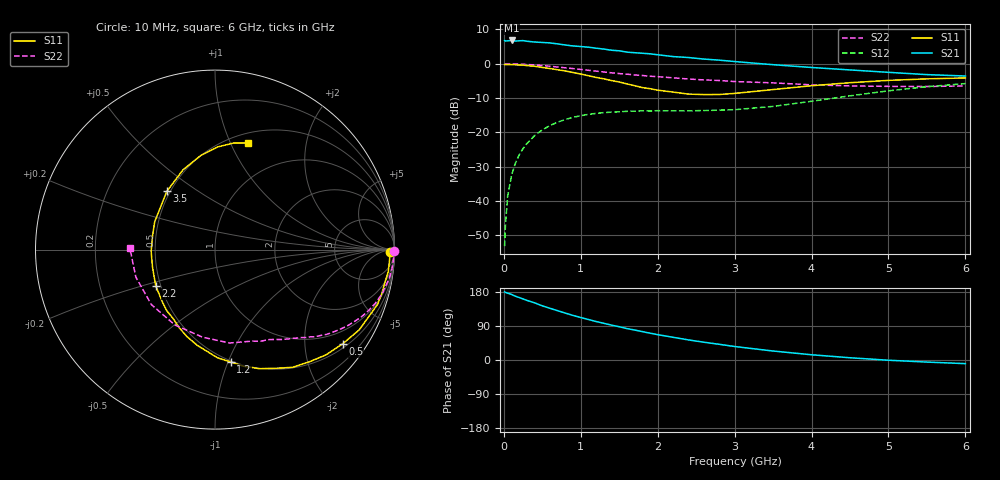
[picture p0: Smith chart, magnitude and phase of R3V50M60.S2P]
! SIEMENS Small Signal Semiconductors
! BFR181
! Si NPN RF Bipolar Junction Transistor in SOT23
! VCE = 0.5 V  IC = 0.6 mA
! Common Emitter S-Parameters:  May  1996
# GHz  S  MA  R  50
!  f  S11  S21  S12  S22
! GHz  MAG  ANG  MAG  ANG  MAG  ANG  MAG  ANG
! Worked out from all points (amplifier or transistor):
!   36 points, 10 MHz to 6 GHz, reference 50 ohm
!   highest |S21| = 6.8 dB at 100 MHz (marker M1)
!   |S21| within 3 dB of that: start of sweep to 1.491 GHz
!   unconditionally stable (mu >= 1): 2.116 GHz to 4.796 GHz; 5.83 GHz to end of sweep
!   at 250 MHz: K = 0.14, MSG = 15.7 dB, |S12| = -24.7 dB
!   at 1.4 GHz: K = 0.70, MSG = 9.0 dB, |S12| = -14.1 dB
!   at 6 GHz: K = 1.00, MAG = 0.7 dB, |S12| = -5.8 dB
!   S11 on the Smith chart (normalised r, x): 10 MHz: 58, -30; 500 MHz: 0.61, -2.93; 1.2 GHz: 0.49, -1.02; 2.2 GHz: 0.47, -0.22; 3.5 GHz: 0.48, +0.38; 6 GHz: 0.60, +1.16
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0.01  0.9732 -0.8  2.181 179.7  0.0022 96.5  0.998 -0.3
0.02  0.9747 -1.5  2.149 178.5  0.0043 90.7  0.9875 -0.7
0.05  0.9741 -3.7  2.157 176.4  0.0119 87.6  0.9974 -1.9
0.1  0.9733 -7.3  2.186 173.0  0.0236 85.8  0.9948 -3.8
0.15  0.9644 -10.8  2.141 168.3  0.0355 81.6  0.9922 -5.9
0.25  0.9558 -18.6  2.177 161.1  0.0583 76.7  0.9839 -9.5
0.5  0.8842 -36.4  2.044 142.9  0.1089 65.3  0.9426 -18.4
0.6  0.8522 -43.5  2.013 136.4  0.1261 60.5  0.9199 -21.7
0.7  0.8171 -49.9  1.946 130.1  0.1412 56.4  0.8968 -24.8
0.9  0.7452 -62.5  1.817 117.6  0.1661 49.0  0.8505 -30.0
1.1  0.6697 -76.1  1.744 106.8  0.183 42.8  0.8036 -34.8
1.2  0.6321 -82.1  1.686 101.5  0.1893 39.7  0.7811 -37.2
1.5  0.5425 -100.5  1.545 87.8  0.1994 33.6  0.7192 -42.5
1.6  0.5087 -108.0  1.477 82.9  0.2029 32.1  0.7052 -44.0
1.9  0.4337 -128.3  1.396 70.8  0.2052 28.8  0.6582 -48.7
2.2  0.387 -148.6  1.273 59.9  0.2062 27.5  0.6238 -53.4
2.4  0.3615 -164.5  1.233 53.0  0.2059 27.9  0.5997 -56.6
2.8  0.3565 167.1  1.129 41.4  0.211 30.1  0.5703 -63.7
3.5  0.421 129.6  0.969 23.7  0.2393 35.8  0.5269 -81.0
4.5  0.5298 98.7  0.813 5.9  0.341 37.2  0.4759 -117.9
5.5  0.6027 80.1  0.695 -5.5  0.4636 26.3  0.4667 -160.8
6  0.6218 72.9  0.663 -9.6  0.514 18.8  0.4751 178.7
